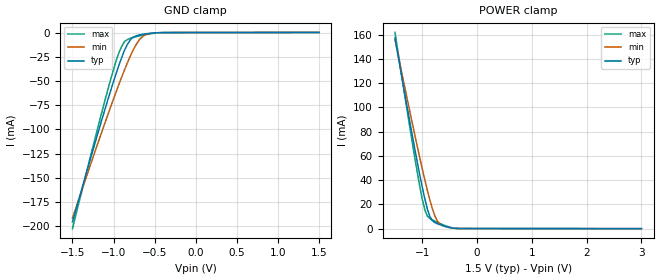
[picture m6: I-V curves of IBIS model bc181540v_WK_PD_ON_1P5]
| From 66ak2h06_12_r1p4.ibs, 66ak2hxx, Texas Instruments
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|   Model Cell bc181540v_WK_PD_ON_1P5
|bc181540v_WK_PD_ON_1P5
[Model]   bc181540v_WK_PD_ON_1P5
Model_type   Input
Polarity   Non-Inverting
Vinl =  0.525
Vinh =  0.975
C_comp   1.17072p   0.570099p   1.17447p
[Model Spec]
Vinl   0.525   0.4725   0.5775
Vinh   0.975   0.8775   1.0725
[Temperature Range]   25   125   -40
[Voltage Range]   1.5   1.35   1.65
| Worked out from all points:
|   GND clamp passes 1 mA (typ) near -0.58 V on its own axis
|   POWER clamp passes 1 mA (typ) near -0.51 V on its own axis
[POWER_clamp]
|   voltage   I(typ)   I(min)   I(max)
-1.5V     157.3mA    155.9mA    161.8mA
-1.227V   87.62mA    96.25mA    83.14mA
-1.045V   43.9mA     58.1mA     34.44mA
-1V       33.82mA    48.99mA    23.94mA
-954.5mV  24.44mA    40.14mA    15.44mA
-909.1mV  16.23mA    31.65mA    10.43mA
-863.6mV  10.07mA    23.72mA    8.413mA
-772.7mV  5.032mA    10.65mA    6.234mA
-727.3mV  4.099mA    6.402mA    5.261mA
-636.4mV  2.628mA    2.64mA     3.445mA
-454.5mV  524.7uA    552.6uA    733.8uA
3V        0A         0A         0A
[GND_clamp]
|   voltage   I(typ)   I(min)   I(max)
-1.5V     -195.7mA   -191.7mA   -202.7mA
-1.227V   -114.7mA   -123.3mA   -110.2mA
-1.045V   -62.86mA   -79.19mA   -51.5mA
-954.5mV  -38.71mA   -58.01mA   -25.55mA
-893.9mV  -24.33mA   -44.5mA    -13.23mA
-863.6mV  -17.76mA   -37.93mA   -9.063mA
-772.7mV  -5.411mA   -20.03mA   -5.365mA
-681.8mV  -2.38mA    -6.956mA   -3.455mA
-621.2mV  -1.507mA   -2.795mA   -2.343mA
-560.6mV  -834.7uA   -1.052mA   -1.386mA
-348.5mV  -31.63uA   -32.36uA   -47.93uA
1.5V      86.37uA    49.39uA    140.3uA
